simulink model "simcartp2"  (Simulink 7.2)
settings: Solver=ode45  StartTime=0.0  StopTime=50.0  RelTol=1e-3
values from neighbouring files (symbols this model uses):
  A = [0,1,0,0;0,0,-m/M*g,0;0,0,0,1;0,0,g/l*(M+m)/M,0]    [cartp.m]
  B = [0,0;1/M,-1/(l*M);0,0;-1/(M*l),1/l^2*(M+m)/(M*m)]    [cartp.m]
  C = [1,0,0,0;0,0,1,0]    [cartp.m]
  D = zeros(2)    [cartp.m]
  K = Ktot(1:4)    [cartp.m]
  L = -place(A',C(1,:)',roots(pobs))'    [cartp.m]
undefined symbols (not defined in the file or in its folder): Reference

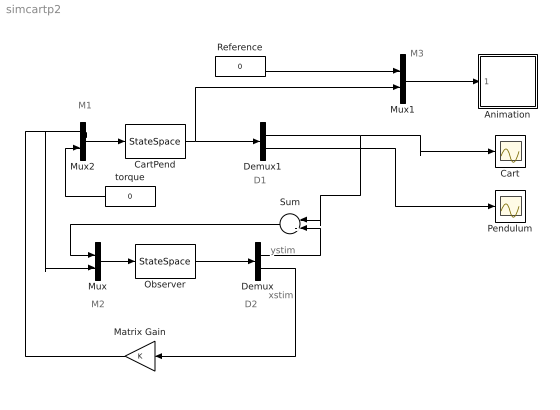
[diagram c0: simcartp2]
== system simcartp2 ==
  note: xstim
  note: ystim
  note: M1
  note: M2
  note: M3
  note: D1
  note: D2
  Animation : Subsystem  mask(Pendulum plot){RefBlock=Reference}
      mask prompts: RefBlock "DC reference signal block name:"
      mask help: Pendulum plot
  Cart : Scope
  CartPend : StateSpace  A=A  B=B  C=C  D=D  X0=[0;0;0.1;0]
  Demux : Demux  Outputs=[1;4]
  Demux1 : Demux  Outputs=2
  Matrix Gain : Gain  Orientation=left  Gain=K  Multiplication=Matrix(K*u)
  Mux : Mux  Inputs=2
  Mux1 : Mux  Inputs=[1;2]
  Mux2 : Mux  Inputs=2
  Observer : StateSpace  A=A  B=[L,B(:,1)]  C=[C(1,:);eye(4)]  D=zeros(5,2)  X0=[0;0;0;0]
  Pendulum : Scope
  Reference : Constant  Value=0
  Sum : Sum  Orientation=left  Inputs=|-|+
  torque : Constant  Orientation=left  Value=0
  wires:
  Observer/1 -> Demux/1
  Demux/1 -> Sum/2
  Mux/1 -> Observer/1
  Sum/1 -> Mux/1
  Mux2/1 -> CartPend/1
  Mux1/1 -> Animation/1(in_1)
  CartPend/1 -> Mux1/2, Demux1/1
  Demux/2 -> Matrix Gain/1
  Demux1/1 -> Cart/1, Sum/1
  Demux1/2 -> Pendulum/1
  torque/1 -> Mux2/2
  Matrix Gain/1 -> Mux/2, Mux2/1
  Reference/1 -> Mux1/1

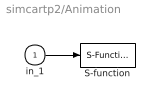
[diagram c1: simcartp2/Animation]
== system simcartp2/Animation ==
  in_1 : Inport
  S-function : S-Function  FunctionName=pendan  Parameters=RefBlock  EnableBusSupport=off
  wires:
  in_1/1 -> S-function/1
